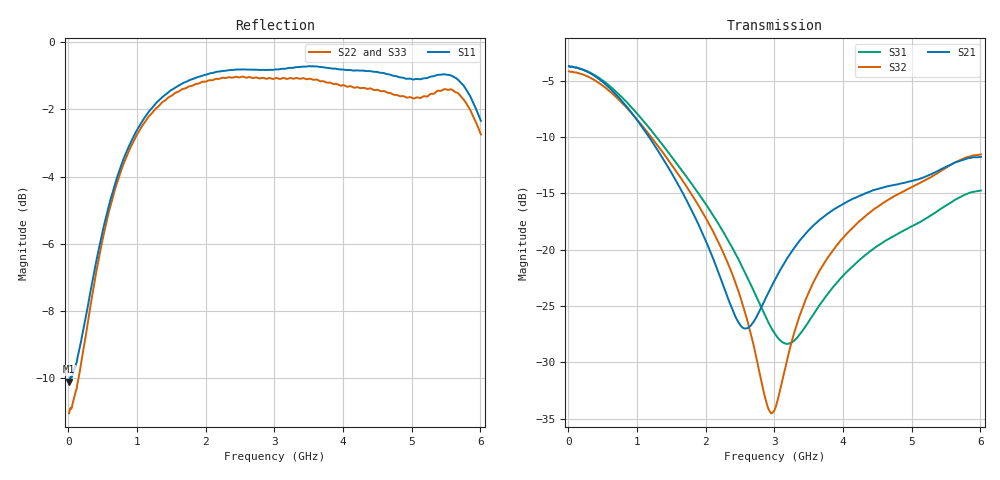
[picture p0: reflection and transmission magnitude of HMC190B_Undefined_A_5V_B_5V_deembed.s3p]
! Device:	HMC190B
! Description:	GaAs MMIC SPDT Reflective Switch
! Package:	8-lead mini small outline package
! Frequency:	DC -  3 GHz
! Ports:
! RFC = Port 1
! RF1 = Port 2
! RF2 = Port 3
! State: Undefined
! Control Voltages:
! A  = 5 V
! B  = 5 V
! Data:	Data was collected using a calibrated network analyzer with AFR software.
!	Fixtures were calculated using AFR and fixturing was applied to collect
!	this Deembedded  S Parameter data of HMC190B.
! Note:	Analog Devices supplies this data as a sample of measured data at the package pin
!	for this product.  Your particular data for this product may vary.
!	Data was taken at 25 degrees C.
!	Analog Devices reserves the right to change this data at anytime.
# Hz S  dB  R 50
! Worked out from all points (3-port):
!   601 points, 10 MHz to 6.01 GHz, reference 50 ohm
!   strongest paths, dB at 10 MHz, 1.51 GHz, 3.01 GHz, 4.51 GHz, 6.01 GHz:
!     S21: -3.7, -13.3, -22.7, -14.6, -11.8
!     S32: -4.2, -12.5, -34.1, -16.2, -11.6
!     S31: -3.7, -11.8, -27.5, -19.6, -14.8
!   lowest |S11| = -10.1 dB at 10 MHz (marker M1), VSWR 1.91, Z = 26.2 - j0.439 ohm
!   |S11| at or under -10 dB: start of sweep to 22.84 MHz
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1e7  -10.10 -178.6  -3.73 -1.2  -3.72 -1.2
     -3.72 -1.2  -11.04 -178.3  -4.17 -1.3
     -3.73 -1.2  -4.18 -1.3  -11.02 -178.3
6.1e8  -4.70 -167.2  -5.72 -45.7  -5.53 -46.5
       -5.72 -45.7  -4.89 -162.8  -6.00 -48.6
       -5.53 -46.5  -6.00 -48.6  -5.00 -162.1
1.37e9  -1.63 164.1  -11.85 -82.7  -10.68 -85.9
        -11.86 -82.7  -1.78 168.5  -11.34 -92.5
        -10.69 -85.9  -11.34 -92.5  -1.84 170.7
2.52e9  -0.81 129.8  -26.81 -55.5  -21.38 -106.7
        -26.82 -55.5  -1.03 133.9  -24.51 -145.5
        -21.38 -106.7  -24.51 -145.5  -1.03 138.4
2.89e9  -0.83 119.4  -24.12 -10.8  -26.16 -93.3
        -24.12 -10.8  -1.09 123.6  -33.70 158.1
        -26.17 -93.3  -33.68 158.0  -1.05 129.3
3.01e9  -0.81 116.0  -22.67 -5.7  -27.46 -82.5
        -22.68 -5.7  -1.08 120.2  -34.13 112.0
        -27.47 -82.5  -34.13 112.0  -1.06 126.4
3.44e9  -0.73 104.4  -18.69 -3.0  -26.94 -36.6
        -18.70 -3.0  -1.08 108.6  -24.70 46.6
        -26.95 -36.6  -24.71 46.6  -1.06 116.4
3.94e9  -0.81 91.4  -16.16 -10.9  -22.72 -22.1
        -16.17 -10.9  -1.27 95.0  -19.38 22.9
        -22.73 -22.1  -19.38 22.9  -1.21 104.9
5.27e9  -1.03 65.4  -13.35 -32.4  -17.00 -36.1
        -13.35 -32.4  -1.55 69.0  -13.61 -16.6
        -17.00 -36.1  -13.61 -16.6  -1.49 77.3
6.01e9  -2.34 62.1  -11.78 -34.4  -14.76 -41.3
        -11.78 -34.4  -2.75 66.2  -11.55 -25.1
        -14.76 -41.3  -11.55 -25.1  -2.83 69.4
